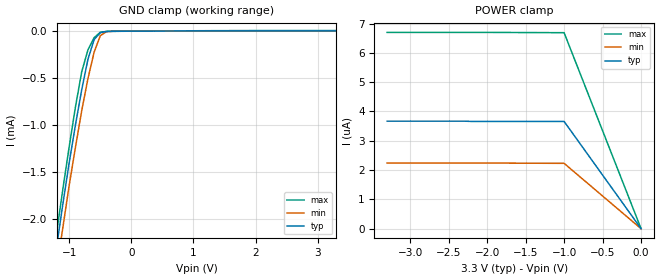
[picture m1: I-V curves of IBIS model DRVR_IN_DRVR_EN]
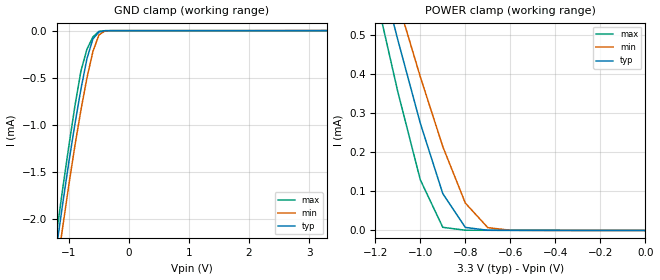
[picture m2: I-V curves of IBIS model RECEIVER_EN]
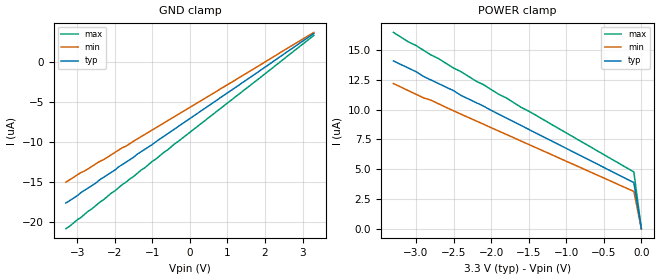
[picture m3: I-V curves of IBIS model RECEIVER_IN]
|   Texas Instruments Incorporated
|   Data Transmissions Products
|   IBIS Model for SN65MLVD203
|   14D SOIC Package
[IBIS Ver]   3.2
[Comment char]   |_char
[File name]   mlvd203.ibs
[File Rev]   2.0
[Date]   21Nov02
[Source]   File originated at Texas Instruments Incorporated.
   Data Transmission Products Group. All data based on
   Simulation Measurements.
[Notes]
[Disclaimer]
(C) Copyright Texas Instruments Incorporated 2002
   All rights reserved
  Texas Instruments Incorporated hereby grants the user of this IBIS
model a non-exclusive, nontransferable license to use this IBIS model
under the following terms.  Before using this IBIS model, the user
should read this license.  If the user does not accept these terms,
the IBIS model should be returned to Texas Instruments within 30 days.
  The user is granted this license only to use the IBIS model and
is not granted rights to sell, load, rent, lease or license the IBIS
model in whole or in part, or in modified form to anyone other than
user.  User may modify the IBIS model to suit its specific applications
but rights to derivative works and such modifications shall belong to
Texas Instruments.
  This IBIS model is provided on an "AS IS" basis and Texas Instruments
makes absolutely no warranty with respect to the information contained
herein.  TEXAS INSTRUMENTS DISCLAIMS AND CUSTOMER WAIVES ALL WARRANTIES,
EXPRESS OR IMPLIED, INCLUDING WARRANTIES OF MERCHANTABILITY OR FITNESS
FOR A PARTICULAR PURPOSE. The entire risk as to quality and performance
is with the Customer. ACCORDINGLY, IN NO EVENT SHALL THE COMPANY BE LIABLE
FOR ANY DAMAGES, WHETHER IN CONTRACT OR TORT,INCLUDING ANY LOST PROFITS
OR OTHER INCIDENTAL, CONSEQUENTIAL, EXEMPLARY, OR PUNITIVE DAMAGES ARISING
OUT OF THE USE OR APPLICATION OF THE IBIS model provided in this package.
Further, Texas Instruments reserves the right to discontinue or make changes
without notice to any product herein to improve reliability, function, or
design. Texas Instruments does not convey any license under patent rights
or any other intellectual property rights, including those of third parties.
Contact Texas Instruments at ATTN:DATA TRANSMISSIONS
[Copyright]   Copyright 2002, Texas Instruments, All Rights Reserved
[Component]   SN65MLVD203D
[Manufacturer]  Texas Instruments Incorporated
[Package]
|   typ   min   max
R_pkg   0.031   0.028   0.034
L_pkg   3.109nH   2.462nH   3.889nH
C_pkg   0.473pF   0.363pF   0.628pF
[Pin]   signal_name   model_name   R_pin   L_pin   C_pin
1   NC   NC
2   R   RECEIVER_OUT   0.032   3.188n   0.473p
3   RE   RECEIVER_EN   0.028   2.462n   0.377p
4   DE   DRVR_IN_DRVR_EN   0.031   2.596n   0.363p
5   D   DRVR_IN_DRVR_EN   0.028   2.521n   0.372p
6   GND   GND   0.034   3.250n   0.476p
7   GND   GND   0.034   3.889n   0.628p
8   NC   NC
9   Y   DRIVER_OUT   0.034   3.250n   0.476p
10   Z   DRIVER_OUT   0.028   2.521n   0.372p
11   B   RECEIVER_IN   0.031   2.596n   0.364p
12   A   RECEIVER_IN   0.028   2.462n   0.377p
13   VCC   POWER   0.032   3.188n   0.473p
14   VCC   POWER   0.033   3.854n   0.622p
[Diff_pin]   inv_pin   vdiff   tdelay_typ   tdelay_min   tdelay_max
| The 'A' or 'Y' pins are Diff_pins and the 'B' or 'Z' pins are inv_pins
   12   11   0.05   0   0   0
   9   10   0.00   0   0   0
| Models and submodels in the file (5): DRVR_IN_DRVR_EN (Input), RECEIVER_EN (Input), RECEIVER_IN (Input), DRIVER_OUT (3-state), RECEIVER_OUT (3-state)
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|   Driver/Driver Enable Model
[Model]   DRVR_IN_DRVR_EN
Model_type   Input
|Signals   D,DE
Vinh = 2.0
Vinl = 0.8
|   typ   min   max
C_comp   1.0pF   NA   NA
|   typ   min   max
[Temperature Range]   25.0   85   -40
[Voltage range]   3.3V   3.0V   3.6V
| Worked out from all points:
|   GND clamp passes 1 mA (typ) near -0.90 V on its own axis
[GND_clamp]
|   Voltage   I(typ)   I(min)   I(max)
-3.3V     -14.3mA    -13.8mA    -14.9mA
-1.2V     -2.27mA    -2.51mA    -2.12mA
-1.1V     -1.82mA    -2.07mA    -1.66mA
-1V       -1.39mA    -1.63mA    -1.22mA
-900mV    -992uA     -1.23mA    -800uA
-800mV    -621uA     -844uA     -431uA
-700mV    -299uA     -504uA     -199uA
-600mV    -88.7uA    -222uA     -68.8uA
-500mV    -15.9uA    -47.1uA    -10.1uA
-400mV    -2.37uA    -4.7uA     -2.62uA
-300mV    -1.1uA     -932nA     -1.79uA
3.3V      3.66uA     2.23uA     6.68uA
[Power_clamp]
| Note that the[POWER_clamp]voltage table is referenced to Vcc
| and is calculated using Vtable=Vcc - Vmeasured.
|   Voltage   I(typ)   I(min)   I(max)
-3.3V     3.67uA     2.24uA     6.7uA
-2V       3.66uA     2.24uA     6.7uA
-1V       3.66uA     2.23uA     6.69uA
0V        0A         0A         0A
|   Receiver Enable Model
[Model]   RECEIVER_EN
Model_type   Input
|Signals   RE
Vinh = 2.0
Vinl = 0.8
|   typ   min   max
C_comp   1.0pF   NA   NA
|   typ   min   max
[Temperature Range]   25.0   85   -40
[Voltage range]   3.3V   3.0V   3.6V
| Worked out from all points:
|   GND clamp passes 1 mA (typ) near -0.90 V on its own axis
|   POWER clamp passes 1 mA (typ) near -1.32 V on its own axis
[GND_clamp]
|   Voltage   I(typ)   I(min)   I(max)
-3.3V     -14.3mA    -13.8mA    -14.9mA
-1.2V     -2.27mA    -2.51mA    -2.12mA
-1.1V     -1.82mA    -2.07mA    -1.66mA
-1V       -1.39mA    -1.63mA    -1.22mA
-900mV    -991uA     -1.22mA    -799uA
-800mV    -621uA     -843uA     -429uA
-700mV    -298uA     -503uA     -198uA
-600mV    -87.7uA    -221uA     -67uA
-500mV    -14.9uA    -46.5uA    -7.98uA
-400mV    -1.52uA    -4.17uA    -1.02uA
-300mV    -611nA     -639nA     -827nA
3.3V      64.2pA     131nA      -188nA
[Power_clamp]
| Note that the[POWER_clamp]voltage table is referenced to Vcc
| and is calculated using Vtable=Vcc - Vmeasured.
|   Voltage   I(typ)   I(min)   I(max)
-3.3V     5.83mA     5.29mA     6.46mA
-1.2V     714uA      787uA      610uA
-1.1V     489uA      587uA      356uA
-1V       275uA      394uA      130uA
-900mV    94.4uA     215uA      8.06uA
-800mV    7.83uA     70.3uA     643nA
-700mV    564nA      7.24uA     510nA
-600mV    340nA      574nA      435nA
0V        64.2pA     165pA      63.7pA
|   Receiver Input Model
[Model]   RECEIVER_IN
Model_type   Input
|Signals   A,B
Vinl = 1.15V
Vinh = 1.35V
|   typ   min   max
C_comp   1.0pF   NA   NA
|   typ   min   max
[Temperature Range]   25.0   85   -40
[Voltage range]   3.3V   3.0V   3.6V
[GND_clamp]
|   Voltage   I(typ)   I(min)   I(max)
-3.3V     -17.6uA    -15uA      -20.8uA
-1.8V     -12.8uA    -10.7uA    -15.3uA
-1.5V     -11.9uA    -9.89uA    -14.3uA
-1.4V     -11.5uA    -9.61uA    -13.9uA
-1V       -10.3uA    -8.48uA    -12.4uA
3.3V      3.55uA     3.69uA     3.31uA
[Power_clamp]
| Note that the[POWER_clamp]voltage table is referenced to Vcc
| and is calculated using Vtable=Vcc - Vmeasured.
|   Voltage   I(typ)   I(min)   I(max)
-3.3V     14.1uA     12.2uA     16.5uA
-3.1V     13.5uA     11.6uA     15.7uA
-3V       13.2uA     11.3uA     15.4uA
-2.9V     12.8uA     11uA       15uA
-2.8V     12.5uA     10.8uA     14.6uA
-2.7V     12.2uA     10.5uA     14.3uA
-2.5V     11.6uA     9.91uA     13.5uA
-2.4V     11.2uA     9.62uA     13.2uA
-2.2V     10.6uA     9.06uA     12.4uA
-1.6V     8.67uA     7.36uA     10.2uA
-100mV    3.87uA     3.13uA     4.77uA
0V        0A         0A         0A
